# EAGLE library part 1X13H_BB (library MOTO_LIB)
1x13 1 mm paste through hole, 1 mm top Ring, 0.1 mm bottom Ring
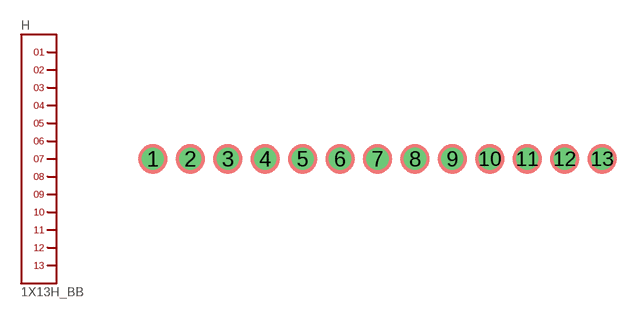
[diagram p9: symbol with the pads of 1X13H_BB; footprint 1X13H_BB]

Designator prefix H

## 1X13H_BB  [1X13H_BB]
1  1
2  2
3  3
4  4
5  5
6  6
7  7
8  8
9  9
10  10
11  11
12  12
13  13

## Footprint 1X13H_BB (pad centres in mm)
Test pin, Through hole, gold pated
drill 1 pad 1.2: 1 0,0; 2 2.54,0; 3 5.08,0; 4 7.62,0; 5 10.16,0; 6 12.7,0; 7 15.24,0; 8 17.78,0; 9 20.32,0; 10 22.86,0; 11 25.4,0; 12 27.94,0; 13 30.48,0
